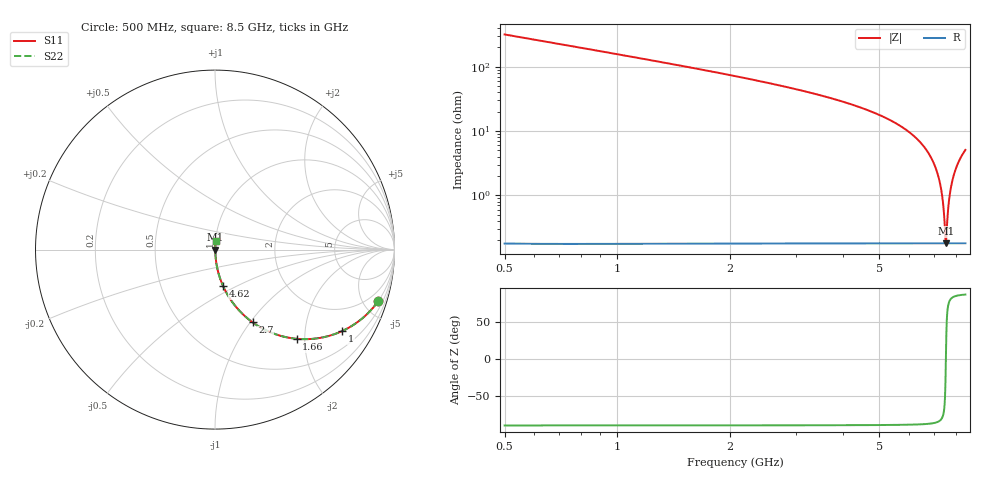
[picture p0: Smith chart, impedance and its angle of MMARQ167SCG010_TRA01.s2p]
! MMARQ167SCG010_TRA01  S-PARAMETER MODEL  ( General Type )
! Model Generated by TAIYO YUDEN Corporation (http://www.ty-top.com)
! Version 1.0
! TAIYO YUDEN Control No. 150305
! Copyright(c) 2015 TAIYO YUDEN CO.,LTD. All Rights Reserved.
! Product Description (link to TY-COMPAS)
! https://ds.yuden.co.jp/TYCOMPAS/or/detail?pn=MMARQ167SCG010BTRA01&u=M
! Products Name : Multilayer Ceramic Capacitors
! Characteristics :
!  Capacitance : 1 pF , Rated Voltage : 250V , TCC : CG / C0G
!  Case Size : 1.6 x 0.8 / 0.063 x 0.031 [mm/inch] , Thickness : 0.7 / 0.028 [mm/inch]
!  (Conditions: Temperature = 25 degC , DC Bias Current/Voltage = 0A / 0V)
! External Node Assignments :
!  1  o---| |---o  2
! GND o---------o GND
! Frequency Range : 500MHz  -  8.5GHz  [ 401 STEP ]
# MHz S RI R 50
! Freq[MHz].  S11 Real  S11 Imag  S21 Real  S21 Imag  S12 Real  S12 Imag  S22 Real  S22 Imag
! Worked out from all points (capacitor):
!   401 points, 500 MHz to 8.5 GHz, reference 50 ohm
!   read as one part in series: C = 1 pF near 540 MHz
!   lowest |Z| = 179 mohm at 7.54 GHz (marker M1)
!   series resonance near 7.539 GHz, so ESL is about 450 pH
!   S11 on the Smith chart (normalised r, x): 500 MHz: 1.00, -6.34; 1 GHz: 1.00, -3.13; 1.66 GHz: 1.00, -1.82; 2.7 GHz: 1.00, -1.03; 4.62 GHz: 1.00, -0.43; 8.5 GHz: 1.00, +0.10
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500  0.9092 -0.287  0.0908 0.287  0.0908 0.287  0.9092 -0.287
1000  0.7093 -0.4535  0.2907 0.4535  0.2907 0.4535  0.7093 -0.4535
1660  0.4541 -0.4969  0.5459 0.4969  0.5459 0.4969  0.4541 -0.4969
1840  0.3982 -0.4884  0.6018 0.4884  0.6018 0.4884  0.3982 -0.4884
2700  0.2096 -0.4053  0.7904 0.4053  0.7904 0.4053  0.2096 -0.4053
3180  0.1457 -0.3507  0.8543 0.3507  0.8543 0.3507  0.1457 -0.3507
4500  0.0508 -0.2156  0.9492 0.2156  0.9492 0.2156  0.0508 -0.2156
4620  0.0457 -0.2048  0.9543 0.2048  0.9543 0.2048  0.0457 -0.2048
5840  0.0135 -0.1073  0.9865 0.1073  0.9865 0.1073  0.0135 -0.1073
6680  0.00439 -0.0509  0.9956 0.0509  0.9956 0.0509  0.00439 -0.0509
6960  0.00292 -0.0336  0.9971 0.0336  0.9971 0.0336  0.00292 -0.0336
7180  0.00221 -0.0205  0.9978 0.0205  0.9978 0.0205  0.00221 -0.0205
7300  0.00197 -0.0135  0.998 0.0135  0.998 0.0135  0.00197 -0.0135
7380  0.00187 -0.00896  0.9981 0.00896  0.9981 0.00896  0.00187 -0.00896
7440  0.00182 -0.00555  0.9982 0.00555  0.9982 0.00555  0.00182 -0.00555
7500  0.00179 -0.00218  0.9982 0.00218  0.9982 0.00218  0.00179 -0.00218
7540  0.00179 5.97e-05  0.9982 -5.97e-05  0.9982 -5.97e-05  0.00179 5.97e-05
7580  0.00179 0.00228  0.9982 -0.00228  0.9982 -0.00228  0.00179 0.00228
7680  0.00185 0.0078  0.9981 -0.0078  0.9981 -0.0078  0.00185 0.0078
7840  0.00206 0.0165  0.9979 -0.0165  0.9979 -0.0165  0.00206 0.0165
8120  0.00277 0.0312  0.9972 -0.0312  0.9972 -0.0312  0.00277 0.0312
8500  0.00435 0.0504  0.9957 -0.0504  0.9957 -0.0504  0.00435 0.0504
